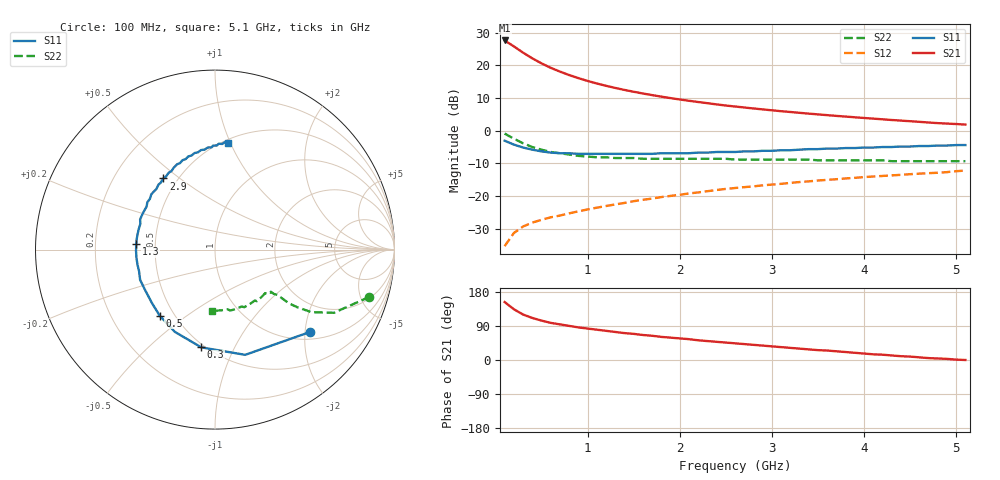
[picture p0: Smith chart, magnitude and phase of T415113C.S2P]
!AT-41511
!S-PARAMETERS at Vce=2.7V  Ic=10mA.  LAST UPDATED 03-28-94
# ghz s ma r 50
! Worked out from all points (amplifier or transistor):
!   51 points, 100 MHz to 5.1 GHz, reference 50 ohm
!   highest |S21| = 27.6 dB at 100 MHz (marker M1)
!   |S21| within 3 dB of that: start of sweep to 262.2 MHz
!   unconditionally stable (mu >= 1): 1.148 GHz to 3.999 GHz; 4.007 GHz to 4.12 GHz; 4.248 GHz to 4.361 GHz
!   at 900 MHz: K = 0.92, MSG = 20.4 dB, |S12| = -24.7 dB
!   at 2.6 GHz: K = 1.09, MAG = 10.6 dB, |S12| = -17.6 dB
!   at 5.1 GHz: K = 0.95, MSG = 7.0 dB, |S12| = -12.3 dB
!   lowest NFmin = 1.10 dB at 100 MHz
!   S11 on the Smith chart (normalised r, x): 100 MHz: 1.18, -2.12; 300 MHz: 0.48, -0.75; 500 MHz: 0.42, -0.40; 1.3 GHz: 0.39, +0.03; 2.9 GHz: 0.42, +0.44; 5.1 GHz: 0.53, +0.98
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0.1  0.7 -41.0  23.95 153.0  0.017 71.0  0.9 -17.0
0.2  0.61 -74.0  19.45 134.0  0.027 60.0  0.75 -28.0
0.3  0.55 -98.0  15.6 120.0  0.034 54.0  0.64 -33.0
0.4  0.51 -116.0  12.75 111.0  0.039 52.0  0.56 -35.0
0.5  0.48 -130.0  10.69 104.0  0.043 51.0  0.51 -36.0
0.6  0.46 -140.0  9.138 98.0  0.047 51.0  0.47 -36.0
0.7  0.45 -150.0  7.996 94.0  0.05 52.0  0.45 -36.0
0.8  0.45 -158.0  7.079 90.0  0.054 53.0  0.43 -36.0
0.9  0.44 -164.0  6.352 86.0  0.058 54.0  0.41 -37.0
1  0.44 -169.0  5.753 83.0  0.062 54.0  0.4 -37.0
1.1  0.44 -174.0  5.258 80.0  0.066 55.0  0.39 -37.0
1.3  0.44 176.0  4.495 74.0  0.074 55.0  0.38 -39.0
1.4  0.44 172.0  4.19 71.0  0.078 56.0  0.38 -39.0
1.6  0.44 165.0  3.693 66.0  0.087 56.0  0.37 -41.0
1.8  0.45 158.0  3.308 61.0  0.096 56.0  0.37 -43.0
2.2  0.46 145.0  2.737 52.0  0.113 55.0  0.37 -47.0
2.6  0.47 134.0  2.335 44.0  0.132 53.0  0.36 -52.0
2.9  0.49 126.0  2.11 38.0  0.145 51.0  0.36 -56.0
3.5  0.52 112.0  1.769 26.0  0.172 48.0  0.35 -65.0
4.3  0.56 96.0  1.452 12.0  0.206 42.0  0.34 -78.0
4.7  0.58 89.0  1.329 5.0  0.223 39.0  0.34 -85.0
5.1  0.6 83.0  1.236 0.0  0.244 36.0  0.34 -93.0
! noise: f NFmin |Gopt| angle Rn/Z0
0.1  1.1  0.21  10  0.2
0.9  1.3  0.22  77  0.16
1.8  1.6  0.25  160  0.12
2.4  1.8  0.36  -170  0.09
